VAR_GLOBAL
	iData1:REAL;
	iData2:INT;
	iData3:STRING;
	
	iData4: WSTRING;
END_VAR
 

VAR_GLOBAL
	gCSV_Buffer: ARRAY[0..MAX_CSV_RING_BUFFER] OF ST_Buffer;
END_VAR

VAR_GLOBAL CONSTANT
	MAX_CSV_ROWS 			: UDINT := 3000;(*最大行数(任务周期为20ms)即10分钟的buffer*)
	MAX_CSV_COLUMNS 		: UDINT := 100;(*最大列数*)
	MAX_CSV_FIELD_LENGTH	: UDINT := 35;(*每个字段的字符长度*)
	MAX_CSV_RING_BUFFER		: UDINT := 4;
END_VAR
